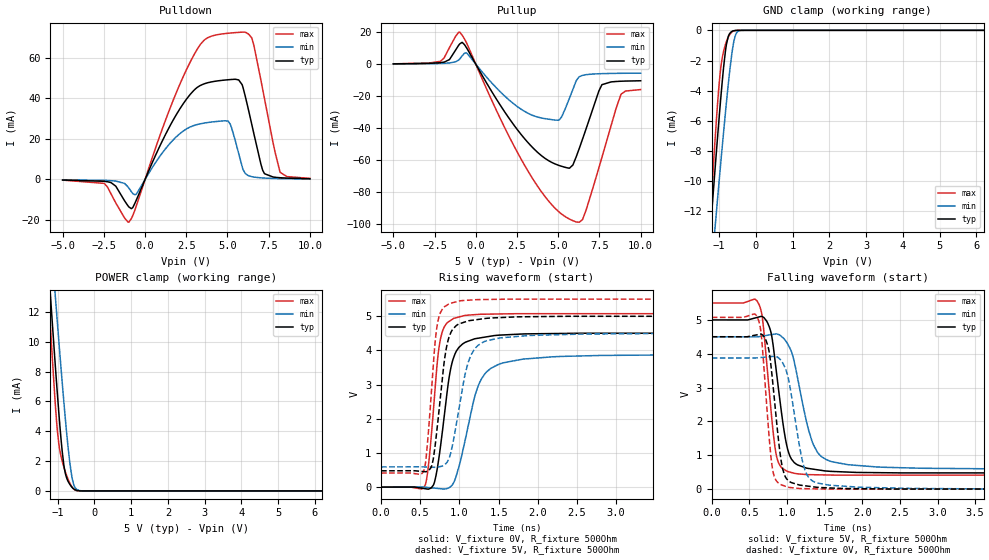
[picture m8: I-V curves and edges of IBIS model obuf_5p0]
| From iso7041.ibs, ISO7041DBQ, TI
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|   obuf_5p0 Model
[Model]   obuf_5p0
Model_type   3-state
Polarity   Non-Inverting
Vmeas = 2.5
Vref = 0
Cref = 2pF
Rref = 100000
|   typ   min   max
C_comp   0.434pF   0.405pF   0.489pF
| Where Nom  PVT is Nominal Process, 5.0V, 27C
|   Fast PVT is Strong Process,  5.5V, -55C
|   Slow PVT is Weak Process,   4.5V, 150C
[Voltage Range]   5   4.5   5.5
|Junction Temperature
[Temperature Range]   27   150   -55
[Pullup Reference]   5   4.5   5.5
[Pulldown Reference]   0   0   0
[Power Clamp Reference]   5   4.5   5.5
[GND Clamp Reference]   0   0   0
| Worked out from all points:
|   slope of the pulldown table from 0 to 0.75 V, typ, clamps not added: 53.8 ohm
|   slope of the pullup table from 0 to 0.75 V, typ, clamps not added: 55.8 ohm
|   GND clamp passes 1 mA (typ) near -0.81 V on its own axis
|   POWER clamp passes 1 mA (typ) near -0.77 V on its own axis
|   falling waveform, V_fixture 5V, R_fixture 500Ohm: 20-80 % time 164ps typ, 239ps min, 130ps max; typ from 5 V to 0.477 V
|   rising waveform, V_fixture 0V, R_fixture 500Ohm: 20-80 % time 161ps typ, 253ps min, 116ps max; typ from 0 V to 4.5 V
|   rising waveform, V_fixture 5V, R_fixture 500Ohm: 20-80 % time 137ps typ, 199ps min, 104ps max; typ from 0.477 V to 5 V
|   falling waveform, V_fixture 0V, R_fixture 500Ohm: 20-80 % time 129ps typ, 179ps min, 107ps max; typ from 4.5 V to 0 V
[Pulldown]
|   Voltage   I(typ)   I(min)   I(max)
-5V       -262.2uA   -171.8uA   -322.7uA
-2.465V   -911.6uA   -444uA     -2.003mA
-980mV    -13.57mA   -4.278mA   -21.09mA
-560mV    -10.71mA   -7.385mA   -13.77mA
1.48V     25.97mA    17.51mA    34.41mA
3.16V     45.42mA    27.11mA    64.24mA
5.05V     49.25mA    28.76mA    72.21mA
5.95V     45.17mA    4.887mA    72.77mA
6.475V    27.17mA    1.381mA    69.85mA
7.135V    4.544mA    746.8uA    44.55mA
8.2V      856.5uA    431.3uA    3.5mA
10V       364.9uA    233.9uA    534.6uA
[GND Clamp]
|   Voltage   I(typ)   I(min)   I(max)
-5V       -142mA     -129.1mA   -170.3mA
-1.25V    -13.66mA   -17.03mA   -12.61mA
-1.13V    -9.808mA   -13.63mA   -7.976mA
-1.07V    -7.928mA   -11.94mA   -5.804mA
-950mV    -4.353mA   -8.649mA   -2.389mA
-875mV    -2.382mA   -6.657mA   -1.357mA
-800mV    -918uA     -4.751mA   -734.3uA
-725mV    -260.7uA   -2.989mA   -334uA
-620mV    -38.78uA   -1.013mA   -56.76uA
-530mV    -5.802uA   -186.8uA   -6.534uA
-410mV    -289.2nA   -8.999uA   -152.5nA
10V       0A         0A         0A
[Pullup]
|   Voltage   I(typ)   I(min)   I(max)
-5V       205.6uA    136.9uA    242.9uA
-2.135V   968.7uA    466uA      1.856mA
-980mV    12.68mA    3.214mA    20.14mA
-545mV    10.01mA    6.871mA    12.99mA
2.11V     -35.27mA   -23.24mA   -47.16mA
4V        -57.51mA   -33.77mA   -80.27mA
5.05V     -63.5mA    -35.04mA   -92.67mA
6.1V      -57.86mA   -10.27mA   -98.98mA
6.475V    -47mA      -6.997mA   -97.44mA
7.645V    -12.96mA   -5.919mA   -58.66mA
8.815V    -10.68mA   -5.704mA   -18.76mA
10V       -10.39mA   -5.618mA   -15.91mA
[POWER Clamp]
|   Voltage   I(typ)   I(min)   I(max)
-5V       226mA      164.8mA    297.6mA
-1.25V    15.08mA    19.1mA     13.31mA
-1.145V   11.28mA    15.69mA    8.935mA
-1.07V    8.647mA    13.28mA    6.055mA
-1.055V   8.132mA    12.81mA    5.528mA
-965mV    5.17mA     9.988mA    3.107mA
-875mV    2.643mA    7.265mA    1.991mA
-815mV    1.487mA    5.534mA    1.467mA
-710mV    615.2uA    2.8mA      748uA
-620mV    274.3uA    1.059mA    305.6uA
-500mV    48.2uA     142.5uA    33.5uA
10V       0A         0A         0A
[Ramp]
R_load = 500
|   typ   min   max
dV/dt_r   2.70201/1.60916e-10   2.3257/2.52647e-10   3.04485/1.16109e-10
dV/dt_f   2.71369/1.63602e-10   2.34488/2.39482e-10   3.05242/1.29184e-10
[Falling Waveform]
V_fixture = 5V
V_fixture_min = 4.5V
V_fixture_max = 5.5V
R_fixture = 500Ohm
C_fixture = 0F
|   Time   V(typ)   V(min)   V(max)
0s        5V         4.5V       5.5V
600.7ps   5.072V     4.5V       5.566V
669.4ps   5.1V       4.522V     5.115V
729.4ps   4.964V     4.544V     3.746V
886.2ps   2.967V     4.57V      783.2mV
1.022ns   1.073V     4.232V     513.5mV
1.268ns   617.9mV    1.913V     430.1mV
1.599ns   524.3mV    809.8mV    416.5mV
3.943ns   480.1mV    597.5mV    415mV
100ns     477.2mV    591.9mV    412.6mV
[Rising Waveform]
V_fixture = 0V
V_fixture_min = 0V
V_fixture_max = 0V
R_fixture = 500Ohm
C_fixture = 0F
|   Time   V(typ)   V(min)   V(max)
0s        -48.98nV   30.07nV    -634.4pV
540.4ps   -37.5mV    2.946mV    -23.09mV
592.2ps   -56.22mV   -8.688mV   398mV
666.4ps   54.3mV     -25.64mV   2.19V
760.7ps   1.227V     -47.18mV   4.362V
917.3ps   3.73V      93.77mV    4.92V
1.268ns   4.366V     3.106V     5.056V
1.807ns   4.479V     3.743V     5.072V
3.943ns   4.501V     3.871V     5.072V
100ns     4.503V     3.876V     5.075V
[Rising Waveform]
V_fixture = 5V
V_fixture_min = 4.5V
V_fixture_max = 5.5V
R_fixture = 500Ohm
C_fixture = 0F
|   Time   V(typ)   V(min)   V(max)
0s        477.2mV    591.9mV    412.6mV
547.2ps   454.4mV    591.5mV    486.7mV
592.2ps   467.5mV    587.8mV    1.275V
651.6ps   660.8mV    582.9mV    3.074V
711.6ps   1.642V     582.1mV    4.657V
833.2ps   4.063V     701.2mV    5.31V
1.078ns   4.836V     3.356V     5.462V
1.219ns   4.898V     4.104V     5.483V
3.492ns   4.996V     4.492V     5.497V
100ns     5V         4.5V       5.5V
[Falling Waveform]
|Gnd
V_fixture = 0V
V_fixture_min = 0V
V_fixture_max = 0V
R_fixture = 500Ohm
C_fixture = 0F
|   Time   V(typ)   V(min)   V(max)
0s        4.503V     3.876V     5.075V
600.7ps   4.56V      3.879V     5.101V
657.9ps   4.58V      3.891V     4.556V
744.7ps   4.24V      3.909V     2.041V
817.9ps   2.978V     3.924V     477.3mV
943.3ps   592.8mV    3.726V     112.9mV
1.176ns   118.6mV    1.149V     18.17mV
1.399ns   55.19mV    183.2mV    8.399mV
3.709ns   3.878mV    6.418mV    2.185mV
100ns     -314.8nV   23.76nV    -628.5pV
